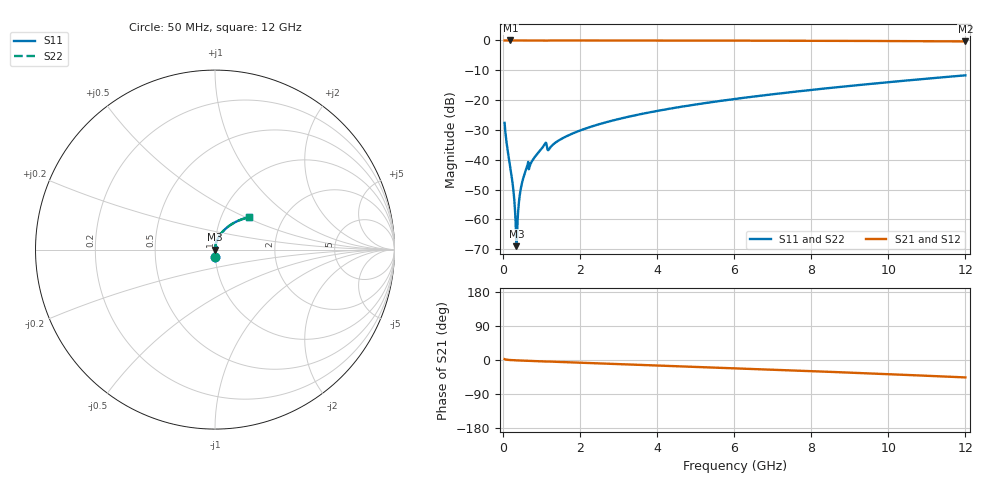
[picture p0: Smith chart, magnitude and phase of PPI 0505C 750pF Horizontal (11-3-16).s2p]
# MHz S MA R 50
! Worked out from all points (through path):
!   1601 points, 50 MHz to 12 GHz, reference 50 ohm
!   highest |S21| = 0.00 dB at 199.4 MHz (marker M1); lowest = -0.3 dB at 12 GHz (marker M2)
!   group delay of S21, straight-line fit = 10.6 ps
!   lowest |S11| = -69.0 dB at 356.2 MHz (marker M3), VSWR 1.00, Z = 50 - j0.0108 ohm
!   |S11| at or under -10 dB: start of sweep to end of sweep
!   |S22| runs from -69.0 to -11.7 dB; largest |S21 - S12| = 0
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50  0.04155 -87.5  0.9989 2.2  0.9989 2.2  0.04155 -87.5
199.375  0.007376 -87.9  0.9997 -0.1  0.9997 -0.1  0.007376 -87.9
266.5938  0.003599 -85.6  0.9997 -0.5  0.9997 -0.5  0.003599 -85.6
318.875  0.001456 -77.8  0.9997 -0.8  0.9997 -0.8  0.001456 -77.8
356.2188  0.0003557 -17.7  0.9996 -0.9  0.9996 -0.9  0.0003557 -17.7
393.5625  0.00114 70.9  0.9996 -1.1  0.9996 -1.1  0.00114 70.9
408.5  0.001573 75.7  0.9996 -1.2  0.9996 -1.2  0.001573 75.7
438.375  0.002416 80.0  0.9996 -1.3  0.9996 -1.3  0.002416 80.0
460.7812  0.003027 81.5  0.9996 -1.4  0.9996 -1.4  0.003027 81.5
542.9375  0.00515 83.7  0.9995 -1.7  0.9995 -1.7  0.00515 83.7
610.1562  0.006913 84.1  0.9995 -2.0  0.9995 -2.0  0.006913 84.1
826.75  0.01099 84.6  0.9994 -2.8  0.9994 -2.8  0.01099 84.6
1080.688  0.01785 80.4  0.998 -3.9  0.998 -3.9  0.01785 80.4
1215.125  0.01543 79.6  0.9981 -4.1  0.9981 -4.1  0.01543 79.6
1506.406  0.02206 83.0  0.999 -5.2  0.999 -5.2  0.02206 83.0
2044.156  0.03156 81.6  0.9987 -7.2  0.9987 -7.2  0.03156 81.6
2910.531  0.04647 78.7  0.998 -10.3  0.998 -10.3  0.04647 78.7
4038.312  0.0664 74.8  0.9967 -14.4  0.9967 -14.4  0.0664 74.8
6025  0.1045 67.7  0.9931 -21.8  0.9931 -21.8  0.1045 67.7
8019.156  0.1484 60.1  0.9872 -29.4  0.9872 -29.4  0.1484 60.1
10013.31  0.1999 52.1  0.9778 -37.5  0.9778 -37.5  0.1999 52.1
12000  0.2602 43.7  0.9632 -46.0  0.9632 -46.0  0.2602 43.7
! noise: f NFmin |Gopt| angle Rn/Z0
50  0.0003087  0.832  0.1726  0.0003876
1372  0.003251  0.6145  3.491  0.001566
2701  0.004651  0.5058  6.532  0.001627
4031  0.006216  0.4646  9.432  0.001946
5360  0.007708  0.4381  12.17  0.002249
6682  0.009166  0.4206  14.74  0.002552
8012  0.01064  0.4096  17.2  0.002871
9341  0.01216  0.4039  19.54  0.00322
1.067e+04  0.01375  0.403  21.81  0.003611
1.2e+04  0.01544  0.4063  24.04  0.004061
